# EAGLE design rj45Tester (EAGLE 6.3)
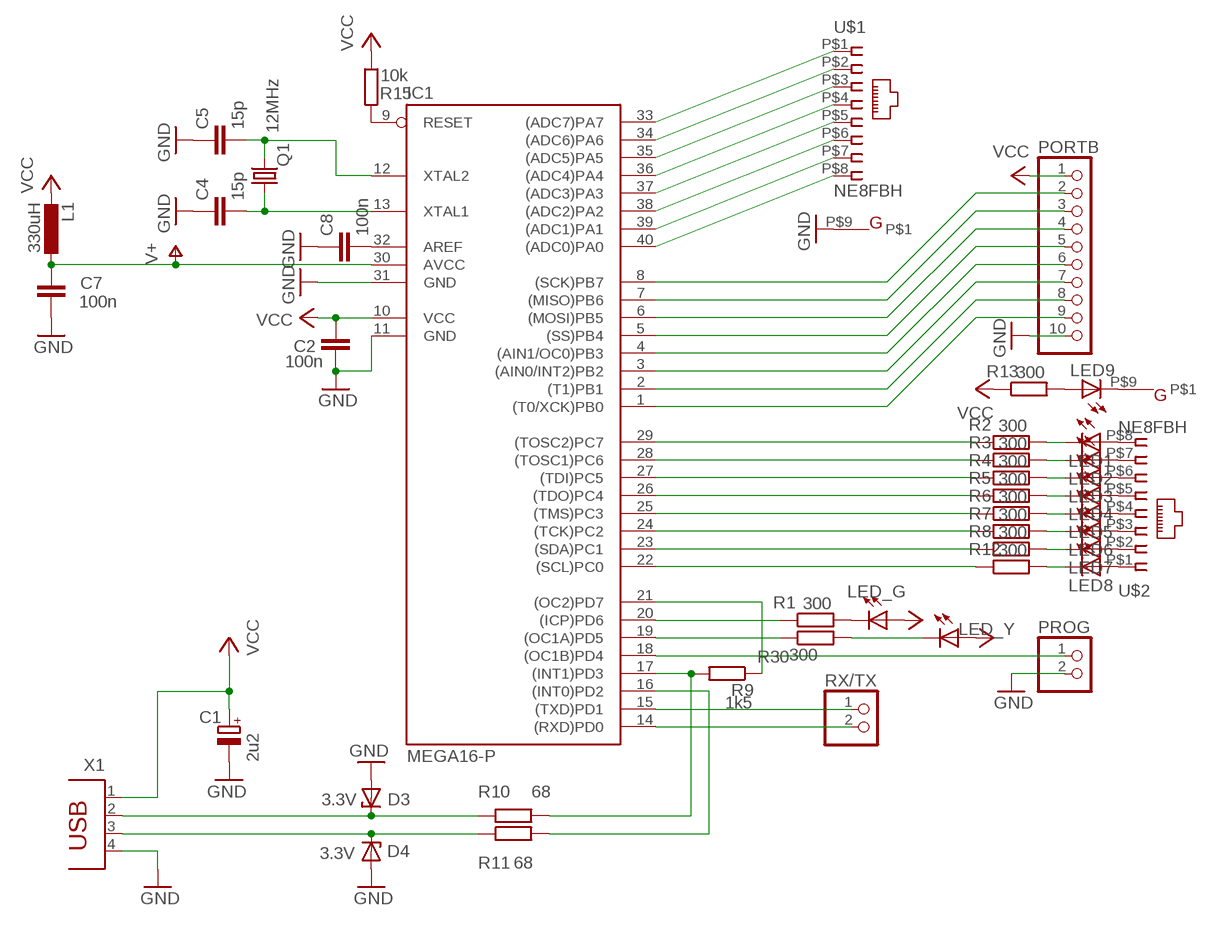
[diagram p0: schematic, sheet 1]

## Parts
C1  2u2  CPOL-EUCT3528  [CT3528]
C2  100n  C-EUC0805  [C0805]
C4  15p  C-EUC1206  [C1206]
C5  15p  C-EUC1206  [C1206]
C7  100n  C-EUC0805  [C0805]
C8  100n  C-EUC0805  [C0805]
D3  3.3V  ZENER-DIODESOD80C  [SOD80C]
D4  3.3V  ZENER-DIODESOD80C  [SOD80C]
IC1  MEGA16-P  [DIL40]
L1  330uH  L-EUL1812  [L1812]
LED1  LEDSMT1206  [1206]
LED2  LEDSMT1206  [1206]
LED3  LEDSMT1206  [1206]
LED4  LEDSMT1206  [1206]
LED5  LEDSMT1206  [1206]
LED6  LEDSMT1206  [1206]
LED7  LEDSMT1206  [1206]
LED8  LEDSMT1206  [1206]
LED9  LEDSMT1206  [1206]
LED_G  LED3MM  [LED3MM]
LED_Y  LED3MM  [LED3MM]
PORTB  10-PIN-SMD-2.54  [10PIN-SMD-2.54]
PROG  PINHD-1X2  [1X02]
Q1  12MHz  CRYTALHC49UP  [HC49UP]
R1  300  R-EU_M1206  [M1206]
R2  300  R-EU_M1206  [M1206]
R3  300  R-EU_M1206  [M1206]
R4  300  R-EU_M1206  [M1206]
R5  300  R-EU_M1206  [M1206]
R6  300  R-EU_M1206  [M1206]
R7  300  R-EU_M1206  [M1206]
R8  300  R-EU_M1206  [M1206]
R9  1k5  R-EU_M1206  [M1206]
R10  68  R-EU_M1206  [M1206]
R11  68  R-EU_M1206  [M1206]
R12  300  R-EU_M1206  [M1206]
R13  300  R-EU_M1206  [M1206]
R15  10k  R-EU_M1206  [M1206]
R30  300  R-EU_M1206  [M1206]
RX/TX  PINHD-1X2  [1X02]
U$1  NE8FBH  [NE8FBH]
U$2  NE8FBH  [NE8FBH]
X1  PN61729  [PN61729]

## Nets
D+: D4.C R11.1 X1.3
D-: D3.C R10.1 X1.2
GND: C1.- C2.2 C4.1 C5.1 C7.2 C8.1 D3.A D4.A IC1.11(GND) IC1.31(GND) PORTB.10 PROG.2 U$1.P$9 X1.4
MISO: IC1.7((MISO)PB6) PORTB.3
MOSI: IC1.6((MOSI)PB5) PORTB.4
N$1: IC1.17((INT1)PD3) R9.2 R10.2
N$2: IC1.9(RESET) R15.1
N$3: IC1.15((TXD)PD1) RX/TX.1
N$4: IC1.14((RXD)PD0) RX/TX.2
N$5: IC1.33((ADC7)PA7) U$1.P$1
N$6: C4.2 IC1.13(XTAL1) Q1.1
N$7: IC1.20((ICP)PD6) R1.1
N$8: IC1.19((OC1A)PD5) R30.1
N$9: LED_G.K(C) R1.2
N$10: IC1.18((OC1B)PD4) PROG.1
N$11: C8.2 IC1.32(AREF)
N$12: IC1.34((ADC6)PA6) U$1.P$2
N$13: IC1.21((OC2)PD7) R9.1
N$14: LED_Y.K(C) R30.2
N$15: IC1.35((ADC5)PA5) U$1.P$3
N$16: IC1.36((ADC4)PA4) U$1.P$4
N$17: IC1.37((ADC3)PA3) U$1.P$5
N$18: IC1.38((ADC2)PA2) U$1.P$6
N$19: IC1.39((ADC1)PA1) U$1.P$7
N$20: IC1.40((ADC0)PA0) U$1.P$8
N$21: LED1.C R2.2
N$22: LED2.C R3.2
N$23: IC1.4((AIN1/OC0)PB3) PORTB.6
N$24: IC1.3((AIN0/INT2)PB2) PORTB.7
N$25: IC1.2((T1)PB1) PORTB.8
N$26: IC1.1((T0/XCK)PB0) PORTB.9
N$27: IC1.16((INT0)PD2) R11.2
N$28: LED3.C R4.2
N$29: LED4.C R5.2
N$30: LED5.C R6.2
N$31: LED6.C R7.2
N$32: LED7.C R8.2
N$33: LED8.C R12.2
N$34: LED1.A U$2.P$8
N$35: LED2.A U$2.P$7
N$36: LED3.A U$2.P$6
N$37: LED4.A U$2.P$5
N$38: C5.2 IC1.12(XTAL2) Q1.2
N$39: LED5.A U$2.P$4
N$40: LED6.A U$2.P$3
N$41: LED7.A U$2.P$2
N$42: LED8.A U$2.P$1
N$43: IC1.29((TOSC2)PC7) R2.1
N$44: IC1.28((TOSC1)PC6) R3.1
N$45: IC1.27((TDI)PC5) R4.1
N$46: IC1.26((TDO)PC4) R5.1
N$47: IC1.25((TMS)PC3) R6.1
N$48: IC1.24((TCK)PC2) R7.1
N$49: IC1.23((SDA)PC1) R8.1
N$50: IC1.22((SCL)PC0) R12.1
N$51: LED9.C U$2.P$9
N$52: LED9.A R13.2
SCK: IC1.8((SCK)PB7) PORTB.2
SS: IC1.5((SS)PB4) PORTB.5
V+: C7.1 IC1.30(AVCC) L1.1
VCC: C1.+ C2.1 IC1.10(VCC) L1.2 LED_G.A LED_Y.A PORTB.1 R13.1 R15.2 X1.1

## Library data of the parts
C1 = rcl:CPOL-EU: POLARIZED CAPACITOR, European symbol
C2 C4 C5 C7 C8 = rcl:C-EU: CAPACITOR, European symbol
D3 D4 = diode:ZENER-DIODE: Z-Diode
IC1 = atmel:MEGA16-P: MICROCONTROLLER 16 Kbytes FLASH 1 kbytes SRAM 512 bytes EEPROM USART 8-channel 10 bit ADC Source: avr.lbr
L1 = rcl:L-EU: INDUCTOR, European symbol
LED1-LED9 LED_G LED_Y = led:LED: LED
PORTB = anyma-lib:10-PIN-SMD-2.54
PROG RX/TX = pinhead:PINHD-1X2: PIN HEADER
Q1 = crystal:CRYTAL: CRYSTAL
R1-R13 R15 R30 = rcl:R-EU_: RESISTOR, European symbol
U$1 U$2 = ethercon:NE8FBH
X1 = con-berg:PN61729: BERG USB connector

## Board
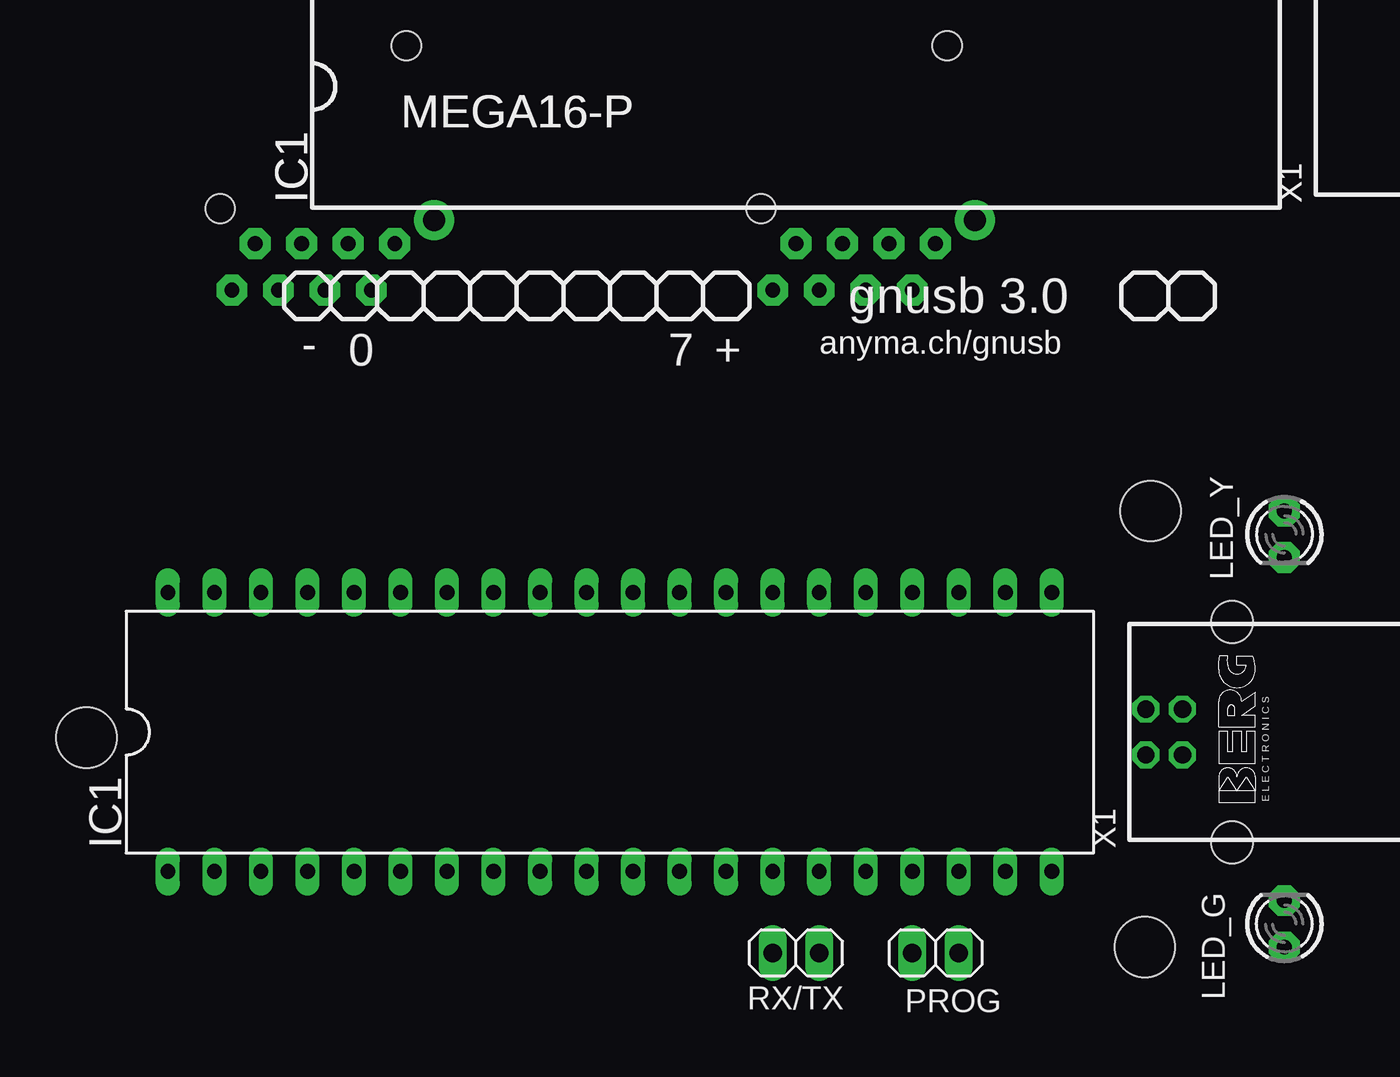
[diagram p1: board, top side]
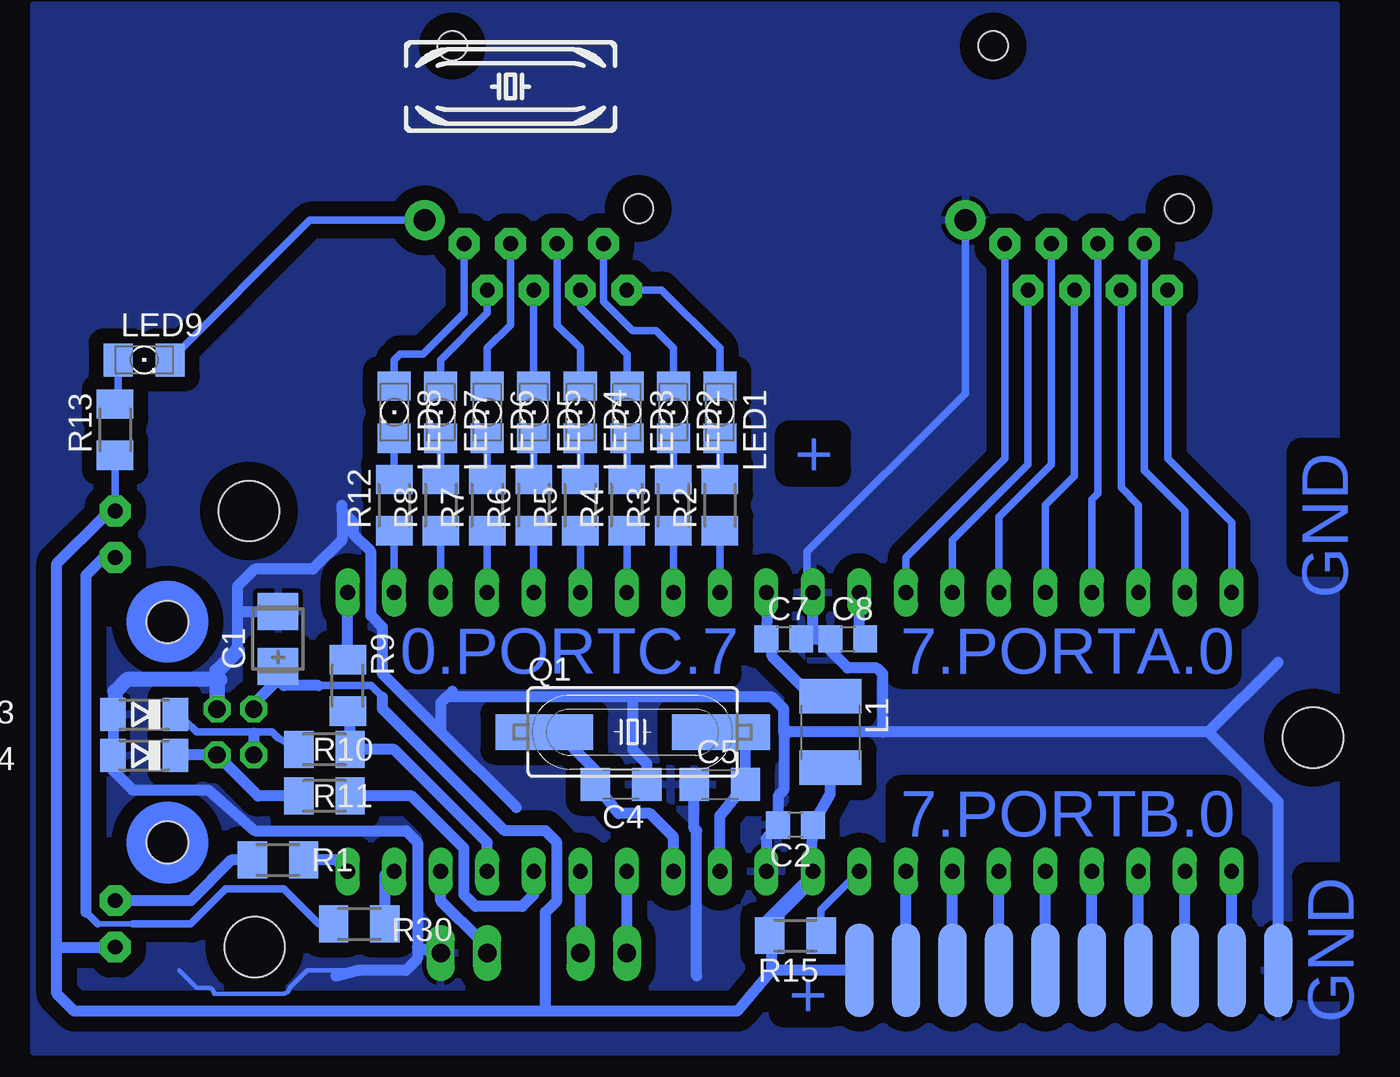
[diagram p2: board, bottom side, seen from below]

No outline drawn. Coordinates in mm, seen from the top.
Copper layers (1*16): Top 0.035mm / dielectric 1.5mm / Bottom 0.035mm
Design rules "10mils": minimum track width 10mil, minimum drill 24mil, track to track 10mil, track to pad 10mil, pad to pad 10mil, via to via 10mil, smd to smd 10mil, copper to edge 40mil, drill to drill 10mil, minimum pad ring 10mil, minimum via ring 8mil, stop-mask expansion 0mil, vias tented up to drill 0mil, thermal gap 10mil
Holes 3.3 mm at 63.18,30.8 62.87,6.99 5.08,18.41

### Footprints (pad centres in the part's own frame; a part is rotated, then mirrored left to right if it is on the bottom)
CT3528 = smd 2 x 2.2: + -1.5,0; - 1.5,0
C0805 = smd 1.3 x 1.5: 1 -0.95,0; 2 0.95,0
C1206 = smd 1.6 x 1.8: 1 -1.4,0; 2 1.4,0
SOD80C = smd 1.4 x 1.8: A 1.7,0; C -1.7,0
DIL40 = drill 0.813 long: 1 -24.13,-7.62; 2 -21.59,-7.62; 3 -19.05,-7.62; 4 -16.51,-7.62; 5 -13.97,-7.62; 6 -11.43,-7.62; 7 -8.89,-7.62; 8 -6.35,-7.62; 9 -3.81,-7.62; 10 -1.27,-7.62; 11 1.27,-7.62; 12 3.81,-7.62; 13 6.35,-7.62; 14 8.89,-7.62; 15 11.43,-7.62; 16 13.97,-7.62; 17 16.51,-7.62; 18 19.05,-7.62; 19 21.59,-7.62; 20 24.13,-7.62; 21 24.13,7.62; 22 21.59,7.62; 23 19.05,7.62; 24 16.51,7.62; 25 13.97,7.62; 26 11.43,7.62; 27 8.89,7.62; 28 6.35,7.62; 29 3.81,7.62; 30 1.27,7.62; 31 -1.27,7.62; 32 -3.81,7.62; 33 -6.35,7.62; 34 -8.89,7.62; 35 -11.43,7.62; 36 -13.97,7.62; 37 -16.51,7.62; 38 -19.05,7.62; 39 -21.59,7.62; 40 -24.13,7.62
L1812 = smd 1.9 x 3.4: 1 -1.95,0; 2 1.95,0
1206 = smd 1.6 x 1.803: A -1.422,0; C 1.422,0
LED3MM = drill 0.813 pad 1.676 octagon: A -1.27,0; K 1.27,0
10PIN-SMD-2.54 = smd 5.08 x 1.524: 1 0,8.89; 2 0,6.35; 3 0,3.81; 4 0,1.27; 5 0,-1.27; 6 0,-3.81; 7 0,-6.35; 8 0,-8.89; 9 0,-11.43; 10 0,-13.97
1X02 = drill 1.016 long: 1 -1.27,0; 2 1.27,0
HC49UP@1 = smd 5.334 x 1.93: 1 -4.826,0; 2 4.826,0
M1206 = smd 1.6 x 2: 1 -1.4,0; 2 1.4,0
NE8FBH = drill 0.8 pad 1.676 octagon: P$1 0,0; P$2 -1.27,-2.54; P$3 -2.54,0; P$4 -3.81,-2.54; P$5 -5.08,0; P$6 -6.35,-2.54; P$7 -7.62,0; P$8 -8.89,-2.54 | drill 1.2 pad 2.184: P$9 2.153,1.267 | hole 1.6: 0.64,10.8; -9.52,1.91
PN61729 = drill 0.95 octagon: 1 1.25,4.71; 2 -1.25,4.71; 3 -1.25,2.71; 4 1.25,2.71 | hole 2.3: -6.02,0; 6.02,0

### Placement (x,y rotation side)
C1  61.59,23.81 90 bottom
C2  33.34,13.65 180 bottom
C4  42.86,15.88 180 bottom
C5  37.47,15.88 0 bottom
C7  33.97,23.81 0 bottom
C8  30.48,23.81 0 bottom
D3  68.9,19.68 180 bottom
D4  68.9,17.46 180 bottom
IC1  33.66,18.73 0 top
L1  31.43,18.73 270 bottom
LED1  37.47,36.2 270 bottom
LED2  40.01,36.2 270 bottom
LED3  42.55,36.2 270 bottom
LED4  45.09,36.2 270 bottom
LED5  47.62,36.2 270 bottom
LED6  50.16,36.2 270 bottom
LED7  52.7,36.2 270 bottom
LED8  55.24,36.2 270 bottom
LED9  68.9,39.05 0 bottom
LED_G  70.48,8.26 90 top
LED_Y  70.48,29.53 270 top
PORTB  20.95,5.71 90 bottom
PROG  51.44,6.67 0 top
Q1  12MHz  [HC49UP@1]  42.23,18.73 0 bottom
R1  61.59,11.75 180 bottom
R2  37.47,31.11 90 bottom
R3  40.01,31.11 90 bottom
R4  42.55,31.11 90 bottom
R5  45.09,31.11 90 bottom
R6  47.62,31.11 90 bottom
R7  50.16,31.11 90 bottom
R8  52.7,31.11 90 bottom
R9  57.78,21.27 270 bottom
R10  59.05,17.78 0 bottom
R11  59.05,15.24 0 bottom
R12  55.24,31.11 90 bottom
R13  70.48,35.24 90 bottom
R15  33.34,7.62 180 bottom
R30  57.15,8.26 180 bottom
RX/TX  43.81,6.67 180 top
U$1  21.91,45.4 0 top
U$2  51.44,45.4 0 top
X1  67.63,18.73 90 top

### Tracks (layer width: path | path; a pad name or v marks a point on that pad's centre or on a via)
D+
  Bottom 0.61: R11.1 62.67,15.24 X1.3 67.18,17.48 D4.C
D-
  Bottom 0.406: R10.1 61.59,18.41 61.91,18.73 62.87,18.73 | 62.87,18.73 66.04,18.73 66.67,19.37 66.88,19.37 D3.C | 62.87,18.73 62.92,18.68
  Bottom 0.61: 62.92,18.68 X1.2
GND
  Bottom 0.254: 57.15,5.71 60.01,5.71 60.96,4.76 arc90 61.28,4.45 65.09,4.45 arc-90 65.41,4.76 66.04,4.76 66.99,5.71
  Bottom 0.406: U$1.P$9 24.06,37.22 32.7,28.57 32.7,26.67 IC1.31
  Bottom 0.61: 10.79,18.73 6.99,22.54 | 10.79,18.73 28.57,18.73 | 28.57,18.73 33.97,18.73 | PORTB.10 6.99,14.92 10.79,18.73 | C8.1 C7.2 32.38,23.81 32.23,23.97 | IC1.31 32.38,24.13 32.23,23.97 | 32.23,23.97 30.48,22.23 28.89,22.23 28.57,21.91 28.57,18.73 | 38.73,15.43 C5.1 38.87,13.46 38.73,13.34 38.73,5.4 | D3.A D4.A 70.6,16.62 69.53,15.56 65.41,15.56 62.87,13.34 54.61,13.34 53.98,12.7 53.98,6.99 | 58.1,30.8 58.1,29.21 59.69,27.62 62.87,27.62 63.82,26.67 63.82,25.4 | 58.1,30.8 58.1,31.11 | C4.1 41.46,17.02 42.23,17.78 42.23,20.64 | 58.1,30.8 57.47,30.16 57.47,29.53 56.52,28.57 56.52,25.08 55.88,24.45 55.88,21.91 52.7,18.73 | IC1.11 34.92,12.91 C2.2 34.29,13.76 34.29,15.24 33.97,15.56 33.97,18.73 | 33.97,18.73 33.97,20 34.61,20.64 42.23,20.64 | 53.98,6.99 53.98,6.35 54.61,5.71 57.15,5.71 58.42,5.4 | 52.7,18.73 52.7,20.32 52.39,20.64 | 52.39,20.64 52.07,20.95 | 42.23,20.64 52.39,20.64 | 52.7,18.73 48.58,14.61 | 53.98,6.99 PROG.2 | 63.82,25.4 63.82,23.18 | C1.- 63.73,25.31 63.82,25.4
  Bottom 0.813: X1.4 64.92,22.08 63.82,23.18 | X1.4 65.07,19.98 | X1.4 64.92,21.44 64.77,21.59 69.85,21.59 70.48,20.95 70.48,19.8 D3.A
  pour Bottom (isolate 0.813): 3.81,1.27 74.93,1.27 74.93,55.88 74.93,58.42 3.81,58.42
MISO
  Bottom 0.61: PORTB.3 IC1.7
MOSI
  Bottom 0.61: PORTB.4 IC1.6
N$1
  Bottom 0.61: IC1.17 50.16,12.7 55.24,17.78 R10.2 57.66,19.74 R9.2
N$2
  Bottom 0.406: R15.1 31.94,9.02 IC1.9
N$3
  Bottom 0.61: RX/TX.1 IC1.15
N$4
  Bottom 0.61: RX/TX.2 IC1.14
N$5
  Bottom 0.406: U$1.P$1 21.91,33.66 27.3,28.26 IC1.33
N$6
  Bottom 0.61: IC1.13 40.01,13.02 41.27,14.29 42.99,14.29 C4.2 44.26,16.64 46.35,18.73 Q1.1
N$7
  Bottom 0.61: R1.1 58.42,11.75 IC1.20
N$8
  Bottom 0.61: R30.1 55.75,10.93 IC1.19
N$9
  Bottom 0.61: LED_G.K 66.36,9.53 64.14,11.75 R1.2
N$10
  Bottom 0.61: IC1.18 52.7,9.53 50.48,7.3 50.48,6.99 PROG.1
N$11
  Bottom 0.406: C8.2 29.84,23.39
  Bottom 0.61: 29.84,23.39 IC1.32
N$12
  Bottom 0.406: U$1.P$2 20.64,33.34 24.77,29.21 IC1.34
N$13
  Bottom 0.61: R9.1 IC1.21
N$14
  Bottom 0.305: 69.53,8.26 71.44,8.26
  Bottom 0.406: R30.2 59.37,8.26 61.28,10.16 64.45,10.16 66.36,8.26 69.53,8.26 | 71.44,8.26 72.07,8.89
  Bottom 0.61: LED_Y.K 71.12,28.26 72.07,27.3 72.07,8.89
N$15
  Bottom 0.406: U$1.P$3 19.37,33.34 22.23,30.48 IC1.35
N$16
  Bottom 0.406: U$1.P$4 18.1,32.7 19.68,31.11 IC1.36
N$17
  Bottom 0.406: U$1.P$5 16.83,31.75 17.14,31.43 IC1.37
N$18
  Bottom 0.406: U$1.P$6 15.56,32.07 14.61,31.11 IC1.38
N$19
  Bottom 0.406: U$1.P$7 14.29,33.02 12.06,30.8 IC1.39
N$20
  Bottom 0.406: U$1.P$8 13.02,33.66 9.53,30.16 IC1.40
N$21
  Bottom 0.406: R2.2 LED1.C
N$22
  Bottom 0.406: R3.2 LED2.C
N$23
  Bottom 0.61: PORTB.6 IC1.4
N$24
  Bottom 0.61: PORTB.7 IC1.3
N$25
  Bottom 0.61: PORTB.8 IC1.2
N$26
  Bottom 0.61: PORTB.9 IC1.1
N$27
  Bottom 0.61: IC1.16 47.62,9.84 48.26,9.21 50.8,9.21 51.44,9.84 51.44,12.38 54.29,15.24 R11.2
N$28
  Bottom 0.406: R4.2 LED3.C
N$29
  Bottom 0.406: R5.2 LED4.C | LED4.C 45.09,34.92 44.77,35.24 44.77,35.09 LED4.C
N$30
  Bottom 0.406: LED5.C R6.2
N$31
  Bottom 0.406: LED6.C R7.2
N$32
  Bottom 0.406: LED7.C R8.2
N$33
  Bottom 0.406: LED8.C R12.2
N$34
  Bottom 0.406: U$2.P$8 40.64,42.86 37.47,39.69 LED1.A
N$35
  Bottom 0.406: U$2.P$7 43.81,42.23 42.23,40.64 40.96,40.64 40.01,39.69 LED2.A
N$36
  Bottom 0.406: U$2.P$6 45.09,41.91 42.55,39.37 LED3.A
N$37
  Bottom 0.406: U$2.P$5 46.35,40.96 45.09,39.69 LED4.A
N$38
  Bottom 0.61: IC1.12 37.47,14.16 C5.2 36.06,18.29 36.51,18.73 Q1.2
N$39
  Bottom 0.406: U$2.P$4 LED5.A
N$40
  Bottom 0.406: U$2.P$3 48.9,40.96 50.16,39.69 LED6.A
N$41
  Bottom 0.406: U$2.P$2 50.16,41.59 52.7,39.05 LED7.A
N$42
  Bottom 0.406: U$2.P$1 51.44,41.59 53.66,39.37 54.93,39.37 55.24,39.05 LED8.A
N$43
  Bottom 0.406: IC1.29 R2.1
N$44
  Bottom 0.406: IC1.28 R3.1
N$45
  Bottom 0.406: IC1.27 R4.1
N$46
  Bottom 0.406: R5.1 IC1.26
N$47
  Bottom 0.406: R6.1 IC1.25 | IC1.25 47.62,26.04 47.94,25.72 47.94,26.04 IC1.25
N$48
  Bottom 0.406: R7.1 IC1.24
N$49
  Bottom 0.406: R8.1 IC1.23
N$50
  Bottom 0.406: R12.1 IC1.22
N$51
  Bottom 0.406: U$2.P$9 59.86,46.67 LED9.C
N$52
  Bottom 0.406: LED9.A 70.32,36.81 R13.2
SCK
  Bottom 0.61: PORTB.2 IC1.8
SS
  Bottom 0.61: PORTB.5 IC1.5
V+
  Bottom 0.61: C7.1 34.82,26.25 IC1.30 | C7.1 34.92,23.71 | L1.1 32.43,20.68 34.61,22.86 34.61,23.6 C7.1
VCC
  Bottom 0.406: 59.37,21.27 56.52,21.27 55.88,20.64 | R13.1 LED_Y.A
  Bottom 0.61: 30.48,5.71 29.53,6.67 | 30.48,5.71 34.61,5.71 | R15.2 34.61,7.49 34.61,5.71 | LED_Y.A 70.8,30.48 71.12,30.48 73.66,27.94 73.66,6.99 | L1.2 31.43,15.34 C2.1 32.49,11.21 IC1.10 | PORTB.1 30.48,5.71 | 34.61,5.71 36.51,3.49 46.99,3.49 | 46.99,3.49 46.99,8.89 46.35,9.53 46.35,12.7 46.99,13.34 49.21,13.34 55.88,20 55.88,20.64 | 46.99,3.49 72.71,3.49 73.66,4.45 73.66,6.99 | 73.66,6.99 LED_G.A | X1.1 62.92,20.27 61.59,21.59 | 61.59,21.59 C1.+ | 59.37,21.27 61.28,21.27 61.59,21.59
  Bottom 0.813: IC1.10 32.38,10.79 34.92,8.26 34.92,7.81 R15.2
(copper drawn outside any net)
  shapes: Bottom circle x2

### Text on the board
Bottom: + | GND | 7.PORTA.0 | 0.PORTC.7 | 7.PORTB.0 | GND | +
tNames: - | 0 | 7 | + | + | 7 | 0 | - | MEGA16-P | MEGA16-P | MEGA16-P | E L E C T R O N I C S | E L E C T R O N I C S | E L E C T R O N I C S | IC1 | IC1 | IC1 | X1 | X1 | gnusb 3.0 | - | 0 | 7 | + | anyma.ch/gnusb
